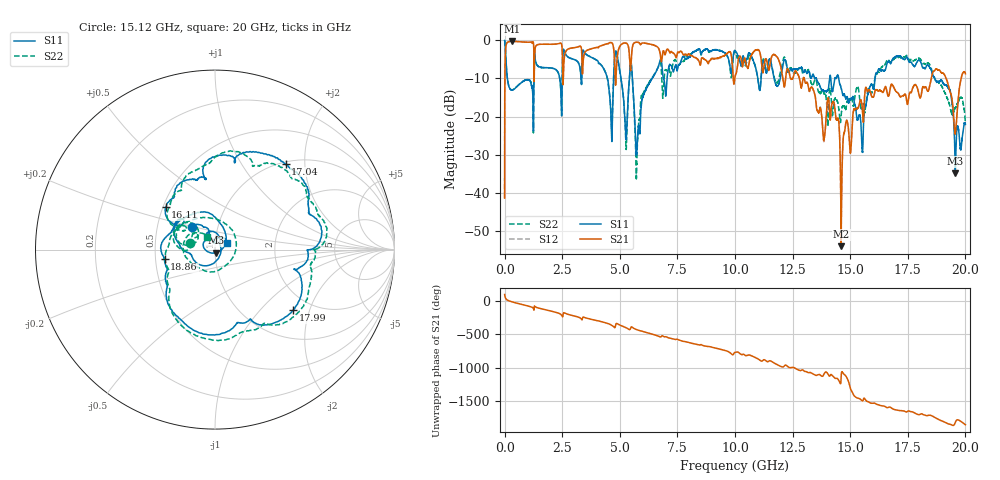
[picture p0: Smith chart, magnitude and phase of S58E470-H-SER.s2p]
!{S58E470}
!Johanson Technology Inc.
!www.johansontechnology.com
!Test Board Conditions:
!Substrate Type  RO4350B
!Substrate Thickness  60 mil
!Substrate Dk  3.66
!TL Type: GCPW
!TL Trace Width  115 mil
!TL Gap  52 mil
!Electrode orientation  Horizontal
!DUT TOPOLOGY	SERIES
!Mounting Pad LxW  55x428 mil
! Created Wed Apr 14 11:50:10 2021
# mhz S ma R 50
! 2 Port Network Data from SP1.SP block
! freq  magS11  angS11  magS21  angS21  magS12  angS12  magS22  angS22
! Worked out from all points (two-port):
!   20001 points, 300 kHz to 20 GHz, reference 50 ohm
!   highest |S21| = -0.23 dB at 315.3 MHz (marker M1); lowest = -54.1 dB at 14.61 GHz (marker M2)
!   |S21| within 3 dB of the highest: 34.17 MHz to 1.269 GHz (1.235 GHz wide, 190 % of centre); 3.48 GHz to 4.752 GHz (1.272 GHz wide, 30.9 % of centre)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
!   lowest |S11| = -35.0 dB at 19.56 GHz (marker M3), VSWR 1.04, Z = 50.4 - j1.74 ohm
!   |S11| at or under -10 dB: 121 MHz to 1.266 GHz (1.145 GHz wide, 165 % of centre); 14.5 GHz to 16.08 GHz (1.574 GHz wide, 10.3 % of centre); 18.67 GHz to end of sweep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
!   |S22| runs from -36.4 to 0.0 dB; largest |S21 - S12| = 0.011
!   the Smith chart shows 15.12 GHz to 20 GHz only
!   S11 on the Smith chart (normalised r, x): 15.12 GHz: 0.75, +0.20; 16.11 GHz: 0.52, +0.28; 17.04 GHz: 1.03, +1.60; 17.99 GHz: 1.61, -1.56; 18.86 GHz: 0.56, -0.06; 20 GHz: 1.15, +0.09
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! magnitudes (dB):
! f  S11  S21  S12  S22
! 300 kHz  0.0  -41.4  -41.4  0.0
! 107.3 MHz  -9.3  -0.6  -0.6  -9.3
! 315.3 MHz  -13.1  -0.2  -0.2  -13.0
! 3.334 GHz  -11.5  -2.2  -2.2  -11.4
! 4.617 GHz  -19.9  -0.6  -0.6  -19.3
! 4.868 GHz  -3.5  -5.8  -5.8  -3.4
! 5.26 GHz  -25.0  -0.7  -0.7  -26.6
! 5.487 GHz  -5.5  -6.5  -6.5  -6.0
! 5.743 GHz  -28.7  -0.5  -0.5  -31.2
! 6.667 GHz  -6.9  -1.9  -1.9  -7.0
! 10 GHz  -2.7  -9.6  -9.6  -3.0
! 13.33 GHz  -9.5  -12.3  -12.3  -11.5
! 14.29 GHz  -11.7  -16.2  -16.1  -16.7
! 14.61 GHz  -12.5  -54.1  -49.3  -19.9
! 15.12 GHz  -14.9  -19.5  -19.4  -16.8
! 16.11 GHz  -8.8  -12.9  -12.9  -9.3
! 16.67 GHz  -5.5  -14.6  -14.6  -5.1
! 17.04 GHz  -4.2  -13.6  -13.6  -4.7
! 17.99 GHz  -5.2  -14.4  -14.4  -4.7
! 18.86 GHz  -10.9  -7.8  -7.8  -11.3
! 19.56 GHz  -35.0  -24.5  -24.5  -17.6
! 20 GHz  -22.1  -8.8  -8.7  -22.0
